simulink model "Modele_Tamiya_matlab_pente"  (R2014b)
settings: Solver=ode15s  StartTime=0.0  StopTime=6  RelTol=1e-3
libraries: fl_lib x15, nesl_utility x5, elec_lib x1

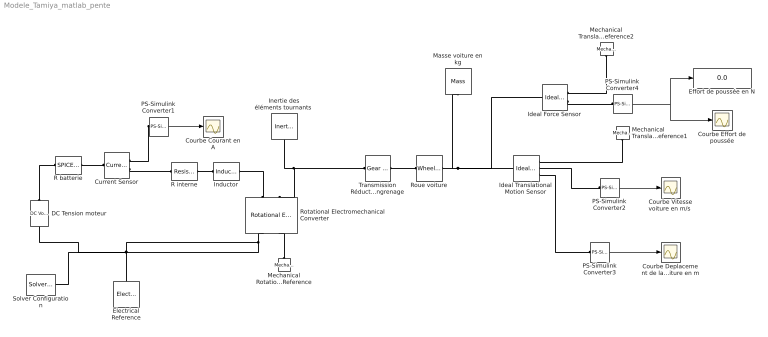
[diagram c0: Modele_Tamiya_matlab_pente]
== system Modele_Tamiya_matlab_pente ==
  "Courbe Vitesse voiture en m/s " : Scope
  Courbe Courant en A : Scope
  Courbe Deplacement de la voiture en m : Scope
  Courbe Effort de poussée : Scope
  Current Sensor : fl_lib/Electrical/Electrical Sensors/Current Sensor
  DC Tension moteur : fl_lib/Electrical/Electrical Sources/DC Voltage Source  v0=0 V
  Effort de poussée en N : Display
  Electrical Reference : fl_lib/Electrical/Electrical Elements/Electrical Reference
  Ideal Force Sensor : fl_lib/Mechanical/Mechanical Sensors/Ideal Force Sensor
  Ideal Translational Motion Sensor : fl_lib/Mechanical/Mechanical Sensors/Ideal Translational Motion Sensor  offset=0 m
  Inductor : fl_lib/Electrical/Electrical Elements/Inductor  l=0.00001 mH  r=0 Ohm  g=1e-9 1/Ohm  i_specify=off  i_priority=High  i=0 A  v_specify=off  v_priority=High  v=0 V  i_L_specify=on  i_L_priority=High  i_L=0 A
  "Inertie des éléments tournants " : fl_lib/Mechanical/Rotational Elements/Inertia  inertia=43.7e-6 kg*m^2  w_specify=on  w_priority=High  w=0 rad/s  t_specify=off  t_priority=High  t=0 N*m
  Masse voiture en kg : fl_lib/Mechanical/Translational Elements/Mass  mass=0 kg  v_specify=on  v_priority=High  v=0 m/s  f_specify=off  f_priority=High  f=0 N
  Mechanical Rotational Reference : fl_lib/Mechanical/Rotational Elements/Mechanical Rotational Reference
  Mechanical Translational Reference1 : fl_lib/Mechanical/Translational Elements/Mechanical Translational Reference
  Mechanical Translational Reference2 : fl_lib/Mechanical/Translational Elements/Mechanical Translational Reference
  PS-Simulink Converter{1..4} (4 alike) : nesl_utility/PS-Simulink Converter  PhysicalDomain=network_engine_domain  SubClassName=ps_output  LeftPortType=input  RightPortType=output  PseudoPeriodic=off  Frequencies=[]  Unit=1  AffineConversion=off
  R batterie : elec_lib/Additional Components/SPICE-Compatible Components/Passive Devices/SPICE Resistor  SCALE=1  R_param=1  R=0.06 Ohm  RSH=0 Ohm  LENGTH=1e-06 m  WIDTH=1e-06 m  NARROW=0 m  T_param=1  TC1=0 1/K  TC2=0 1/K^2  TOFFSET=0 K  TFIXED=300.15 K  TMEAS=300.15 K
  R interne : fl_lib/Electrical/Electrical Elements/Resistor  R=0.19 Ohm  i_specify=off  i_priority=High  i=0 A  v_specify=off  v_priority=High  v=0 V
  Rotational Electromechanical Converter : fl_lib/Electrical/Electrical Elements/Rotational Electromechanical Converter  K=0.006 V/(rad/s)  i_specify=off  i_priority=High  i=0 A  v_specify=off  v_priority=High  v=0 V  t_specify=off  t_priority=High  t=0 N*m  w_specify=off  w_priority=High  w=0 rad/s
  Roue voiture : fl_lib/Mechanical/Mechanisms/Wheel and Axle  R=0.033 m  or=1  orient=1  t_specify=off  t_priority=High  t=0 N*m  f_specify=off  f_priority=High  f=0 N
  Solver Configuration : nesl_utility/Solver Configuration  PhysicalDomain=network_engine_domain  SubClassName=solver  LeftPortType=input  RightPortType=generic  Accelerate=off  Tones=[]  Harmonics=[]  SimulateNoise=off  Profile=off  UseLocalSampling=off  EnableSwitchedLinearOptims=on  FrequencyDomain=off  UseCCode=off  RelTol=0.001  AbsTol=1e-06  MinStep=1e-09  ToWorkspace=off  DoDC=off  ResidualTolerance=1e-9  UseLocalSolver=off  LocalSolverChoice=NE_BACKWARD_EULER_ADVANCER  LocalSolverSampleTime=.001  DoFixedCost=off  MaxNonlinIter=3  MaxModeIter=2  LinearAlgebra=Sparse  DelaysMemoryBudget=1024  AutomaticFiltering=on  FilteringTimeConstant=0.001
  Transmission Réducteur à engrenage : fl_lib/Mechanical/Mechanisms/Gear Box  ratio=8.33  t_in_specify=off  t_in_priority=High  t_in=0 N*m  t_out_specify=off  t_out_priority=High  t_out=0 N*m
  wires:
  PS-Simulink Converter2/1 -> "Courbe Vitesse voiture en m/s "/1
  PS-Simulink Converter1/1 -> Courbe Courant en A/1
  PS-Simulink Converter3/1 -> Courbe Deplacement de la voiture en m/1
  PS-Simulink Converter4/1 -> Effort de poussée en N/1, Courbe Effort de poussée/1
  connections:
  Current Sensor/RConn2 -- R interne/LConn1
  R interne/RConn1 -- Inductor/LConn1
  Rotational Electromechanical Converter/RConn1 -- DC Tension moteur/RConn1 -- Solver Configuration/RConn1 -- Electrical Reference/LConn1
  Rotational Electromechanical Converter/LConn1 -- Inductor/RConn1
  Transmission Réducteur à engrenage/LConn1 -- Rotational Electromechanical Converter/LConn2 -- "Inertie des éléments tournants "/LConn1
  Roue voiture/LConn1 -- Transmission Réducteur à engrenage/RConn1
  R batterie/RConn1 -- Current Sensor/LConn1
  DC Tension moteur/LConn1 -- R batterie/LConn1
  Roue voiture/RConn1 -- Ideal Translational Motion Sensor/LConn1 -- Ideal Force Sensor/LConn1 -- Masse voiture en kg/LConn1
  Ideal Translational Motion Sensor/RConn2 -- PS-Simulink Converter2/LConn1
  Mechanical Translational Reference1/LConn1 -- Ideal Translational Motion Sensor/RConn1
  PS-Simulink Converter1/LConn1 -- Current Sensor/RConn1
  Mechanical Rotational Reference/LConn1 -- Rotational Electromechanical Converter/RConn2
  Ideal Translational Motion Sensor/RConn3 -- PS-Simulink Converter3/LConn1
  Ideal Force Sensor/RConn2 -- PS-Simulink Converter4/LConn1
  Mechanical Translational Reference2/LConn1 -- Ideal Force Sensor/RConn1
